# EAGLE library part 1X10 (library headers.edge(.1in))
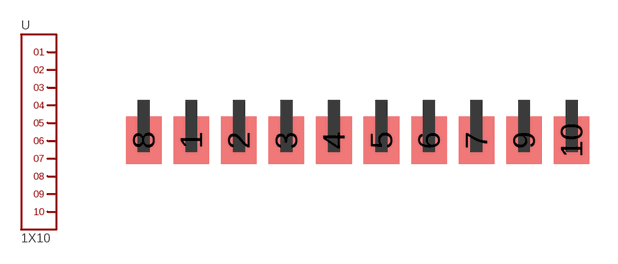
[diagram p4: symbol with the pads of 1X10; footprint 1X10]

Designator prefix -

## 1X10  [1X10]
1  1
2  2
3  3
4  4
5  5
6  6
7  7
8  8
9  9
10  10

## Footprint 1X10 (pad centres in mm)
smd 1.905 x 2.54: 1 2.54,-2.159; 2 5.08,-2.159; 3 7.62,-2.159; 4 10.16,-2.159; 5 12.7,-2.159; 6 15.24,-2.159; 7 17.78,-2.159; 8 0,-2.159; 9 20.32,-2.159; 10 22.86,-2.159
